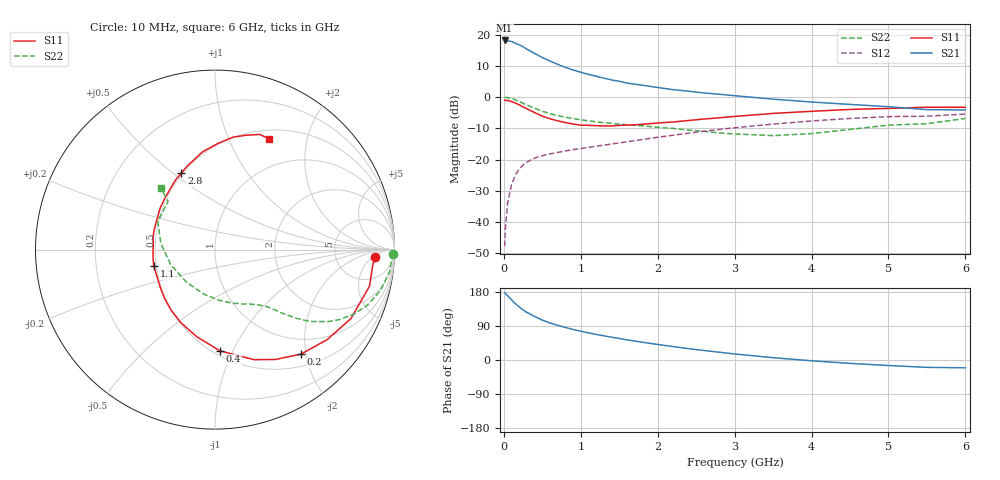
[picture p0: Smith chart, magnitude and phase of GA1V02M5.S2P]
! Infineon Technologies  Discrete & RF Semiconductors
! BF775
! Si NPN RF Bipolar Junction Transistor in SOT23
! VCE = 1 V  IC = 2.5 mA
! Common Emitter S-Parameters:  May  1996
# GHz  S  MA  R  50
!  f  S11  S21  S12  S22
! GHz  MAG  ANG  MAG  ANG  MAG  ANG  MAG  ANG
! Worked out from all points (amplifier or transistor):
!   36 points, 10 MHz to 6 GHz, reference 50 ohm
!   highest |S21| = 18.1 dB at 10 MHz (marker M1)
!   |S21| within 3 dB of that: start of sweep to 314.3 MHz
!   unconditionally stable (mu >= 1): 976 MHz to end of sweep
!   at 250 MHz: K = 0.34, MSG = 18.9 dB, |S12| = -21.7 dB
!   at 1.4 GHz: K = 1.17, MAG = 7.8 dB, |S12| = -15.0 dB
!   at 6 GHz: K = 1.05, MAG = -0.7 dB, |S12| = -5.4 dB
!   S11 on the Smith chart (normalised r, x): 10 MHz: 15, -7; 200 MHz: 0.71, -1.91; 400 MHz: 0.54, -0.89; 1.1 GHz: 0.48, -0.10; 2.8 GHz: 0.49, +0.54; 6 GHz: 0.61, +1.42
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0.01  0.8947 -2.8  8.078 178.1  0.0041 90.2  0.9939 -1.4
0.02  0.8836 -5.3  7.943 175.6  0.008 84.8  0.986 -2.8
0.05  0.8846 -13.3  7.95 169.4  0.0205 81.9  0.9811 -7.2
0.1  0.8494 -26.9  7.785 159.0  0.0396 74.7  0.9488 -14.0
0.15  0.8011 -38.8  7.272 148.7  0.0566 68.1  0.9041 -20.0
0.2  0.754 -50.6  6.88 140.1  0.0705 62.6  0.8536 -24.9
0.25  0.6981 -61.3  6.404 132.2  0.0819 57.6  0.7963 -29.3
0.3  0.6506 -70.5  5.848 125.6  0.0911 54.4  0.747 -32.5
0.4  0.5648 -87.2  5.004 114.9  0.1055 49.0  0.6639 -37.1
0.5  0.4962 -101.7  4.302 105.3  0.1153 45.7  0.5932 -40.2
0.6  0.4506 -114.7  3.784 97.8  0.1234 43.7  0.5419 -42.2
0.7  0.417 -125.9  3.351 91.5  0.1301 42.6  0.5053 -43.9
0.9  0.37 -145.7  2.716 80.6  0.1445 41.7  0.4527 -46.3
1.1  0.3536 -164.8  2.316 71.6  0.1566 42.0  0.4164 -49.2
1.3  0.345 -179.3  2.011 63.8  0.1706 42.3  0.39 -52.0
1.6  0.3565 161.9  1.681 53.1  0.1925 42.6  0.3611 -57.2
2.2  0.3997 134.4  1.317 35.4  0.245 41.4  0.315 -71.9
2.8  0.4664 113.6  1.111 20.5  0.3039 37.5  0.2665 -93.8
3.5  0.5481 97.4  0.928 6.1  0.3699 30.2  0.2413 -131.0
4.5  0.6346 80.8  0.764 -8.9  0.4552 17.5  0.3035 173.6
5.5  0.6883 68.8  0.63 -19.4  0.4951 3.3  0.3748 134.2
6  0.6866 63.8  0.622 -20.6  0.5354 -0.6  0.4556 131.4
